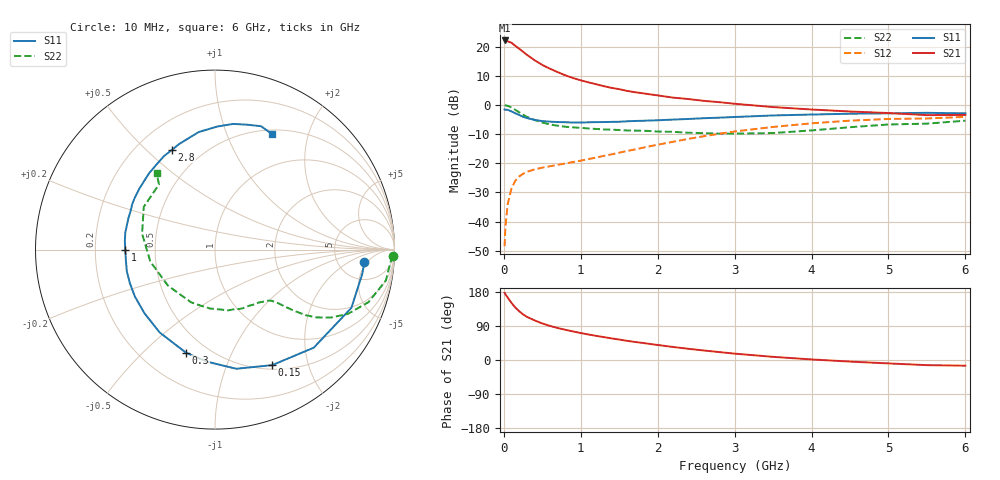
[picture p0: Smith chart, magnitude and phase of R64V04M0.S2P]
! SIEMENS Small Signal Semiconductors
! BFR193
! Si NPN RF Bipolar Junction Transistor in SOT23
! VCE = 4 V  IC = 4 mA
! Common Emitter S-Parameters:  May  1996
# GHz  S  MA  R  50
!  f  S11  S21  S12  S22
! GHz  MAG  ANG  MAG  ANG  MAG  ANG  MAG  ANG
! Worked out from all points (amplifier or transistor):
!   36 points, 10 MHz to 6 GHz, reference 50 ohm
!   highest |S21| = 22.1 dB at 10 MHz (marker M1)
!   |S21| within 3 dB of that: start of sweep to 208 MHz
!   unconditionally stable (mu >= 1): 958.2 MHz to 2.011 GHz
!   at 250 MHz: K = 0.37, MSG = 20.9 dB, |S12| = -23.6 dB
!   at 1.4 GHz: K = 1.08, MAG = 9.7 dB, |S12| = -16.9 dB
!   at 6 GHz: K = 0.97, MSG = 0.3 dB, |S12| = -4.1 dB
!   S11 on the Smith chart (normalised r, x): 10 MHz: 9, -4; 150 MHz: 0.55, -1.46; 300 MHz: 0.38, -0.69; 1 GHz: 0.33, +0.00; 2.8 GHz: 0.34, +0.60; 6 GHz: 0.55, +1.46
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0.01  0.8355 -4.9  12.76 177.1  0.0038 88.8  0.994 -2.0
0.02  0.8312 -9.6  12.65 173.6  0.0081 89.0  0.9803 -4.1
0.05  0.8263 -23.1  12.36 164.7  0.0199 78.2  0.9678 -10.2
0.1  0.7755 -44.8  11.62 150.6  0.0375 68.0  0.9039 -18.9
0.15  0.7182 -63.7  10.3 138.2  0.0504 59.8  0.8228 -25.8
0.2  0.6744 -79.9  9.208 128.6  0.0597 54.1  0.7499 -30.3
0.25  0.6263 -93.9  8.168 120.3  0.0661 50.1  0.6809 -33.7
0.3  0.5971 -105.6  7.243 113.9  0.0715 47.5  0.6257 -35.8
0.4  0.5552 -123.7  5.846 104.5  0.0787 44.9  0.552 -37.9
0.5  0.5296 -137.8  4.852 96.4  0.0843 43.7  0.5004 -39.2
0.6  0.5173 -149.7  4.179 89.9  0.089 44.9  0.4641 -40.2
0.7  0.5099 -158.6  3.655 84.4  0.0942 46.2  0.4407 -41.2
0.8  0.506 -166.1  3.22 79.7  0.0994 47.6  0.4233 -42.3
1  0.4999 180.0  2.643 71.1  0.1111 50.7  0.405 -45.0
1.1  0.5046 174.6  2.44 67.3  0.1183 52.6  0.3961 -47.1
1.6  0.5251 151.7  1.744 50.6  0.1622 58.4  0.3662 -58.6
2.2  0.5617 130.9  1.337 34.4  0.2342 58.7  0.3464 -77.7
2.8  0.6057 113.2  1.117 20.9  0.3209 53.1  0.3223 -104.2
3.5  0.6611 97.9  0.92 8.3  0.4204 42.2  0.3302 -142.6
4.5  0.7077 81.7  0.773 -4.2  0.5387 24.5  0.4158 167.7
5.5  0.7337 69.5  0.67 -13.6  0.587 6.8  0.4787 130.7
6  0.7182 64.0  0.675 -15.0  0.6249 1.7  0.5379 127.2
